(* Logix 5000 Controller export Example_PLC; controller Example_PLC 1769-L32E rev 19.11; software revision 19.01; part 5 of 6 *)
(* tags used below, declared in another part *)
   Incremental : BOOL;   // Position Definition (0=Absolute, 1=Incremental)
   OS_LoadStart : BOOL;
(* AKD_Set_Position, continued *)

ROUTINE Prescan   (* ladder *)
// Prescan
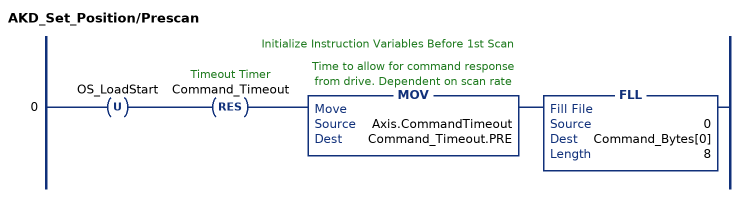
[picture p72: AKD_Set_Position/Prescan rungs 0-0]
   // Initialize Instruction Variables Before 1st Scan
   0: OTU(OS_LoadStart)RES(Command_Timeout)MOV(Axis.CommandTimeout,Command_Timeout.PRE)FLL(0,Command_Bytes[0],8);
END_ROUTINE
END_ADD_ON_INSTRUCTION

ADD_ON_INSTRUCTION AKD_Move_RevB   (* revision 4.1, ExecutePrescan, ExecuteEnableInFalse *)
// Motion Axis Move - Position Move
// Revision note:
// Don't error if Command_Timeout preset is 0
VAR_IN_OUT
   Axis : AKD_Axis; {required}
END_VAR
VAR_INPUT
   Move_Type : SINT; {required}   // Move Type (0=Absolute, 1=Incremental)
   Accel : DINT; {required}   // Acceleration
   Decel : DINT; {required}   // Deceleration
   Speed : DINT; {required}   // Move Speed
   Position : DINT; {required}   // Target Position
END_VAR
VAR_OUTPUT
   DN : BOOL; {access Read Only, visible}   // Command Successfully Initiated
   ER : BOOL; {access Read Only, visible}   // Error
   IP : BOOL; {access Read Only, visible}   // Command in Process
   PC : BOOL; {access Read Only, visible}   // Command Process Complete
END_VAR
VAR
   Step : SINT;   // Sequence Step Number
   Command_Axis_Number : SINT;
   Response_Axis_Number : SINT;
   Set_Accel : AKD_Set_Accel;
   Set_Decel : AKD_Set_Decel;
   Set_Velocity : AKD_Set_Velocity;
   OS_Start_Sequence : BOOL;
   Set_Position : AKD_Set_Position;
   Command_Timeout : TIMER := (PRE := 200);
   Command_Bytes : SINT[64];
   ErrorData : SINT[8];
END_VAR

ROUTINE EnableInFalse   (* ladder *)
// EnableIn_False
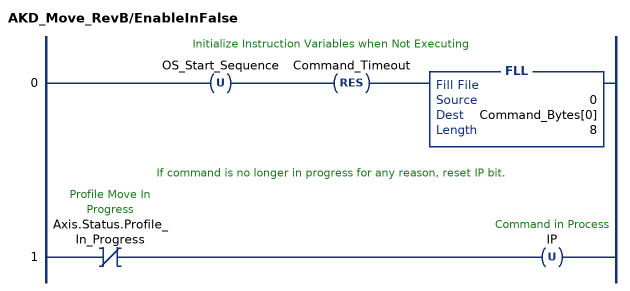
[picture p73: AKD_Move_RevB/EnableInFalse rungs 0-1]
   // Initialize Instruction Variables when Not Executing
   0: OTU(OS_Start_Sequence)RES(Command_Timeout)FLL(0,Command_Bytes[0],8);
   // If command is no longer in progress for any reason, reset IP bit.
   1: XIO(Axis.Status.Profile_In_Progress)OTU(IP);
END_ROUTINE

ROUTINE Logic   (* ladder *)
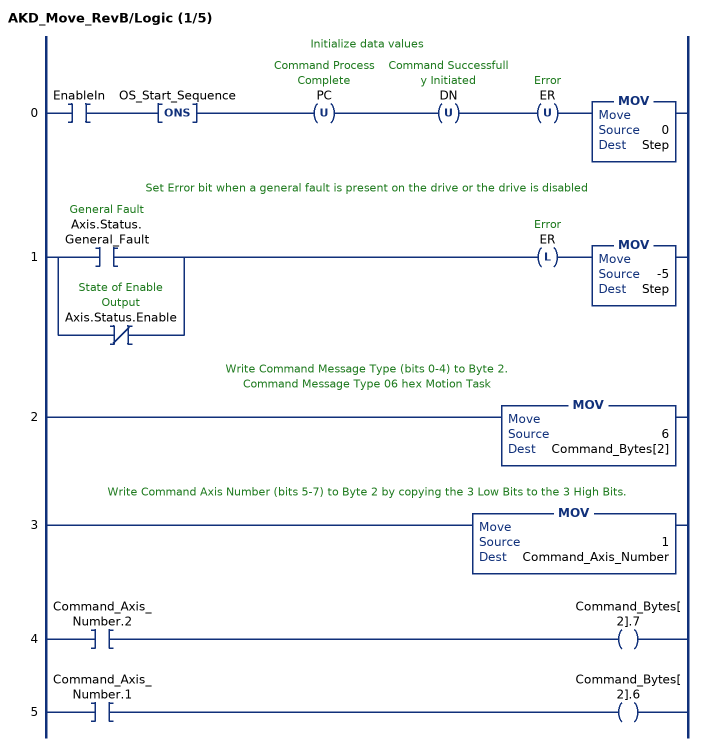
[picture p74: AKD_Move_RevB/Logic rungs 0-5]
   // Initialize data values
   0: XIC(EnableIn)ONS(OS_Start_Sequence)OTU(PC)OTU(DN)OTU(ER)MOV(0,Step);
   // Set Error bit when a general fault is present on the drive or the drive is disabled
   1: [XIC(Axis.Status.General_Fault) ,XIO(Axis.Status.Enable) ]OTL(ER)MOV(-5,Step);
   // Write Command Message Type (bits 0-4) to Byte 2.
   // Command Message Type 06 hex Motion Task
   2: MOV(6,Command_Bytes[2]);
   // Write Command Axis Number (bits 5-7) to Byte 2 by copying the 3 Low Bits to the 3 High Bits.
   3: MOV(1,Command_Axis_Number);
   4: XIC(Command_Axis_Number.2)OTE(Command_Bytes[2].7);
   5: XIC(Command_Axis_Number.1)OTE(Command_Bytes[2].6);
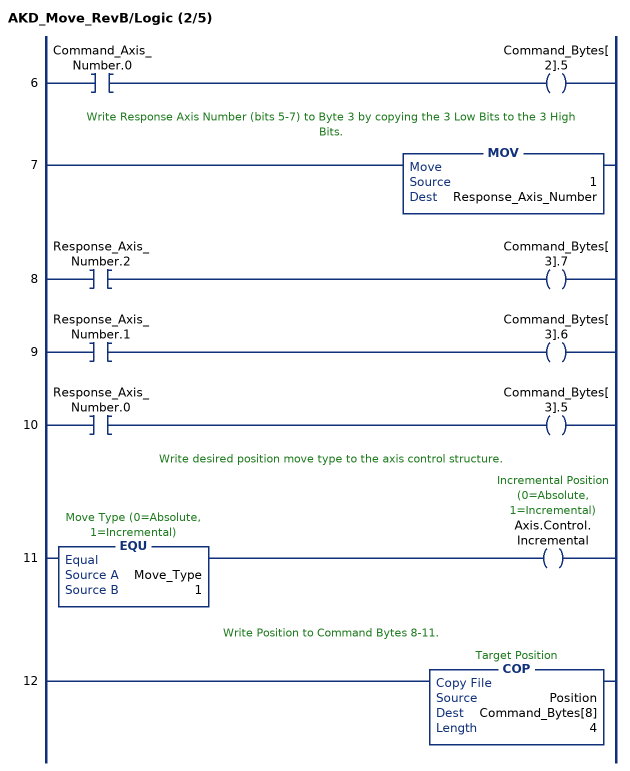
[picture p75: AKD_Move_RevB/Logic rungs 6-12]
   6: XIC(Command_Axis_Number.0)OTE(Command_Bytes[2].5);
   // Write Response Axis Number (bits 5-7) to Byte 3 by copying the 3 Low Bits to the 3 High Bits.
   7: MOV(1,Response_Axis_Number);
   8: XIC(Response_Axis_Number.2)OTE(Command_Bytes[3].7);
   9: XIC(Response_Axis_Number.1)OTE(Command_Bytes[3].6);
   10: XIC(Response_Axis_Number.0)OTE(Command_Bytes[3].5);
   // Write desired position move type to the axis control structure.
   11: EQU(Move_Type,1)OTE(Axis.Control.Incremental);
   // Write Position to Command Bytes 8-11.
   12: COP(Position,Command_Bytes[8],4);
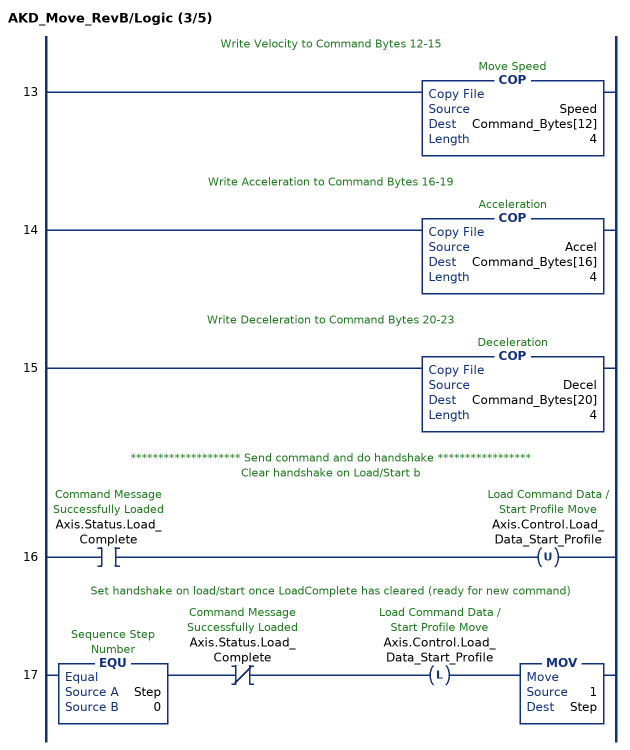
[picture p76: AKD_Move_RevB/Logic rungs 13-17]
   // Write Velocity to Command Bytes 12-15
   13: COP(Speed,Command_Bytes[12],4);
   // Write Acceleration to Command Bytes 16-19
   14: COP(Accel,Command_Bytes[16],4);
   // Write Deceleration to Command Bytes 20-23
   15: COP(Decel,Command_Bytes[20],4);
   // ******************** Send command and do handshake *****************
   // Clear handshake on Load/Start b
   16: XIC(Axis.Status.Load_Complete)OTU(Axis.Control.Load_Data_Start_Profile);
   // Set handshake on load/start once LoadComplete has cleared (ready for new command)
   17: EQU(Step,0)XIO(Axis.Status.Load_Complete)OTL(Axis.Control.Load_Data_Start_Profile)MOV(1,Step);
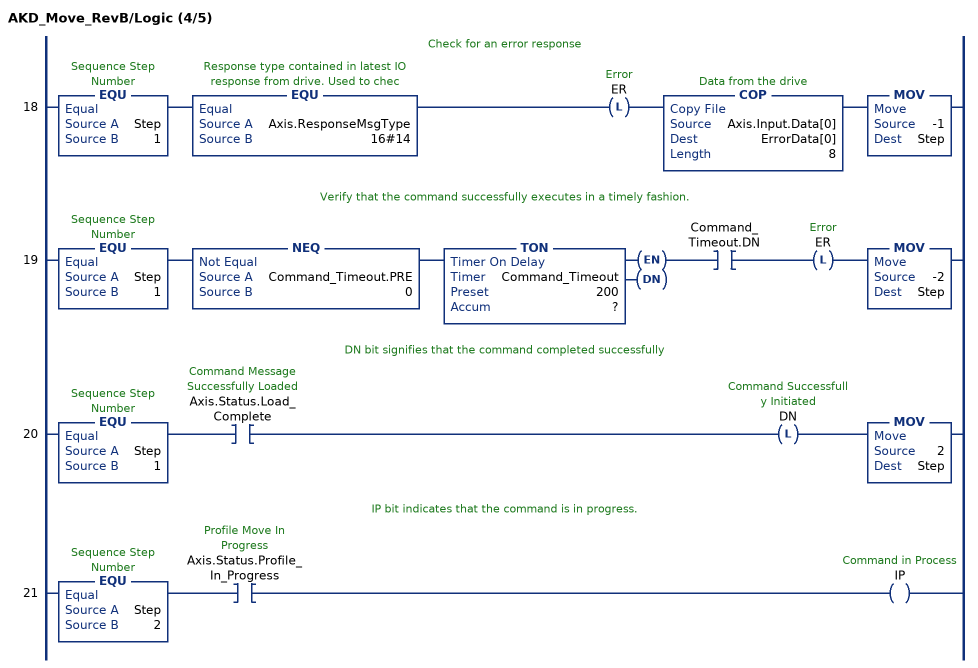
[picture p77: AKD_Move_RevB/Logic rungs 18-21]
   // Check for an error response
   18: EQU(Step,1)EQU(Axis.ResponseMsgType,16#14)OTL(ER)COP(Axis.Input.Data[0],ErrorData[0],8)MOV(-1,Step);
   // Verify that the command successfully executes in a timely fashion.
   19: EQU(Step,1)NEQ(Command_Timeout.PRE,0)TON(Command_Timeout,?,?)XIC(Command_Timeout.DN)OTL(ER)MOV(-2,Step);
   // DN bit signifies that the command completed successfully
   20: EQU(Step,1)XIC(Axis.Status.Load_Complete)OTL(DN)MOV(2,Step);
   // IP bit indicates that the command is in progress.
   21: EQU(Step,2)XIC(Axis.Status.Profile_In_Progress)OTE(IP);
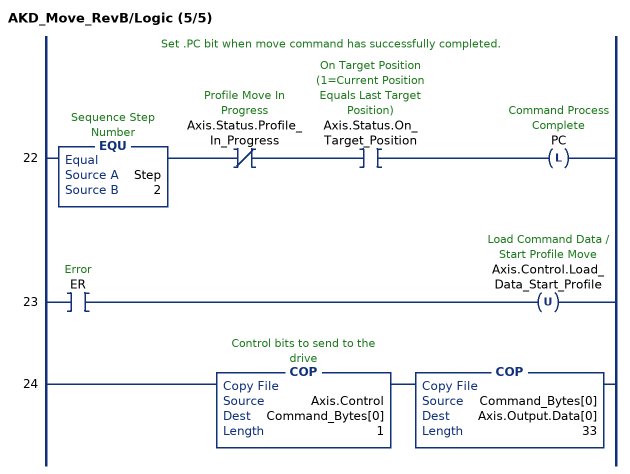
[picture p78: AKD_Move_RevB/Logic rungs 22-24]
   // Set .PC bit when move command has successfully completed.
   22: EQU(Step,2)XIO(Axis.Status.Profile_In_Progress)XIC(Axis.Status.On_Target_Position)OTL(PC);
   23: XIC(ER)OTU(Axis.Control.Load_Data_Start_Profile);
   24: COP(Axis.Control,Command_Bytes[0],1)COP(Command_Bytes[0],Axis.Output.Data[0],33);
END_ROUTINE

ROUTINE Prescan   (* ladder *)
// Prescan
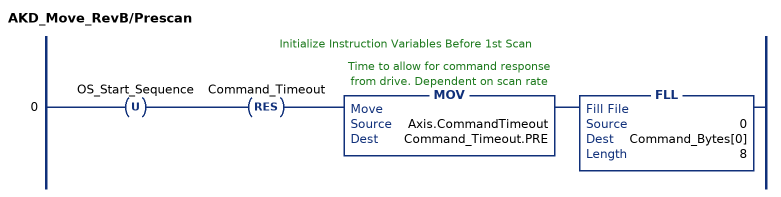
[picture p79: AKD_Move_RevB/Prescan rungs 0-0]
   // Initialize Instruction Variables Before 1st Scan
   0: OTU(OS_Start_Sequence)RES(Command_Timeout)MOV(Axis.CommandTimeout,Command_Timeout.PRE)FLL(0,Command_Bytes[0],8);
END_ROUTINE
END_ADD_ON_INSTRUCTION

ADD_ON_INSTRUCTION AKD_Set_Home_Mode   (* revision 2.0, ExecutePrescan, ExecuteEnableInFalse *)
// Set Homing Mode
VAR_OUTPUT
   DN : BOOL; {access Read Only, visible}   // Command Successful
   ER : BOOL; {access Read Only, visible}   // Error
END_VAR
VAR_IN_OUT
   Axis : AKD_Axis; {required}
END_VAR
VAR_INPUT
   Mode : SINT; {required}   // Home Mode:
END_VAR
VAR
   Command_Bytes : SINT[8];
   Step : DINT;
   Set_Attribute : AKD_Set_Attribute;
END_VAR

ROUTINE EnableInFalse   (* ladder *)
// EnableIn_False
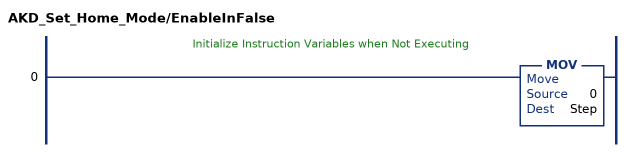
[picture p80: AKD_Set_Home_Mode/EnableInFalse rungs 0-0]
   // Initialize Instruction Variables when Not Executing
   0: MOV(0,Step);
END_ROUTINE

ROUTINE Logic   (* ladder *)
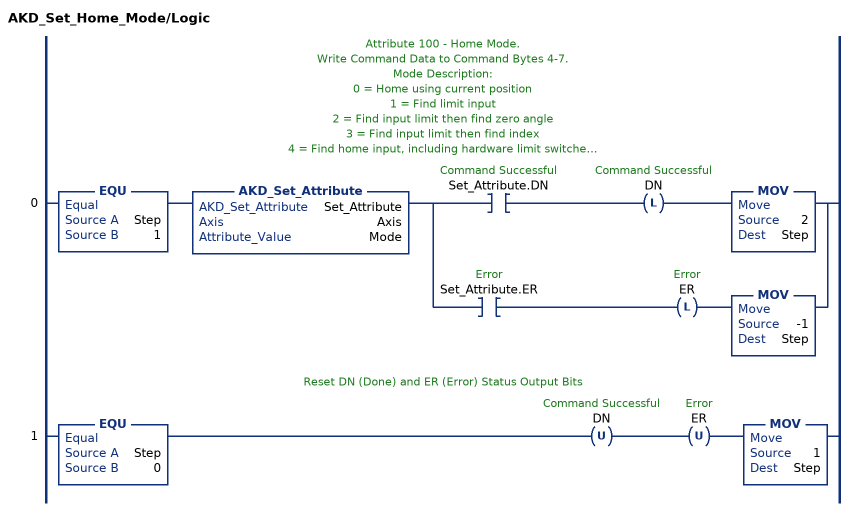
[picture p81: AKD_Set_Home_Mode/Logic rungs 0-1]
   // Attribute 100 - Home Mode.
   // Write Command Data to Command Bytes 4-7.
   // Mode Description:
   // 0 = Home using current position
   // 1 = Find limit input
   // 2 = Find input limit then find zero angle
   // 3 = Find input limit then find index
   // 4 = Find home input, including hardware limit switches
   // 5 = Find home input then find zero angle, including hardware limit switches
   // 6 = Find home input then find index, including hardware limit switches.
   // 7 = Find zero angle
   // 8 = Move until position error exceeded
   // 9 = Move until position error exceeded, then find zero angle
   // 10 = Move until position error exceeded, then find index
   // 11 = Find index signal, without any precondition
   // 12 = Homing to a home-switch, including mechanical stop detection
   0: EQU(Step,1)AKD_Set_Attribute(Set_Attribute,Axis,Mode)[XIC(Set_Attribute.DN) OTL(DN) MOV(2,Step) ,XIC(Set_Attribute.ER) OTL(ER) MOV(-1,Step) ];
   // Reset DN (Done) and ER (Error) Status Output Bits
   1: EQU(Step,0)OTU(DN)OTU(ER)MOV(1,Step);
END_ROUTINE

ROUTINE Prescan   (* ladder *)
// Prescan
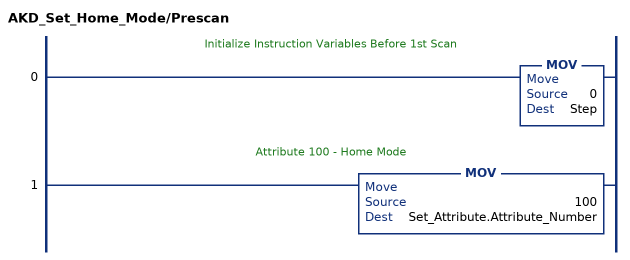
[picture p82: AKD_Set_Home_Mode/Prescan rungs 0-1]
   // Initialize Instruction Variables Before 1st Scan
   0: MOV(0,Step);
   // Attribute 100 - Home Mode
   1: MOV(100,Set_Attribute.Attribute_Number);
END_ROUTINE
END_ADD_ON_INSTRUCTION

ADD_ON_INSTRUCTION AKD_Set_Units   (* revision 2.2, ExecutePrescan, ExecuteEnableInFalse *)
// Set Drive Units for Motion Commands
// Revision note:
// Clean up instruction, especially for error recovery.
VAR_IN_OUT
   Axis : AKD_Axis; {required}
END_VAR
VAR_INPUT
   Units : SINT; {required}   // Drive Units (0=Counts 16 bit)
END_VAR
VAR_OUTPUT
   DN : BOOL; {access Read Only, visible}   // Command Successfully Initiated
   ER : BOOL; {access Read Only, visible}   // Error
END_VAR
VAR
   Set_POSUNIT : AKD_Set_Attribute := (Attribute_Number := 4);
   Set_PROFUNIT : AKD_Set_Attribute := (Attribute_Number := 5);
   Step : SINT;   // Sequence Step Number
   OS_Start_Sequence : BOOL;
   Profile_Ratio : DINT;   // The number of actual feedback counts per second or second2 equal to one velocity or acceleration unit
   Position_Ratio : DINT;   // The number of actual position feedback counts equal to one position unit
   Invalid_Input : BOOL;   // Invalid Units Input
END_VAR

ROUTINE EnableInFalse   (* ladder *)
// EnableIn_False
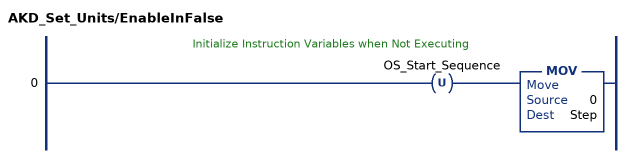
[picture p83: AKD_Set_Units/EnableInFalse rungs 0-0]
   // Initialize Instruction Variables when Not Executing
   0: OTU(OS_Start_Sequence)MOV(0,Step);
END_ROUTINE

ROUTINE Logic   (* ladder *)
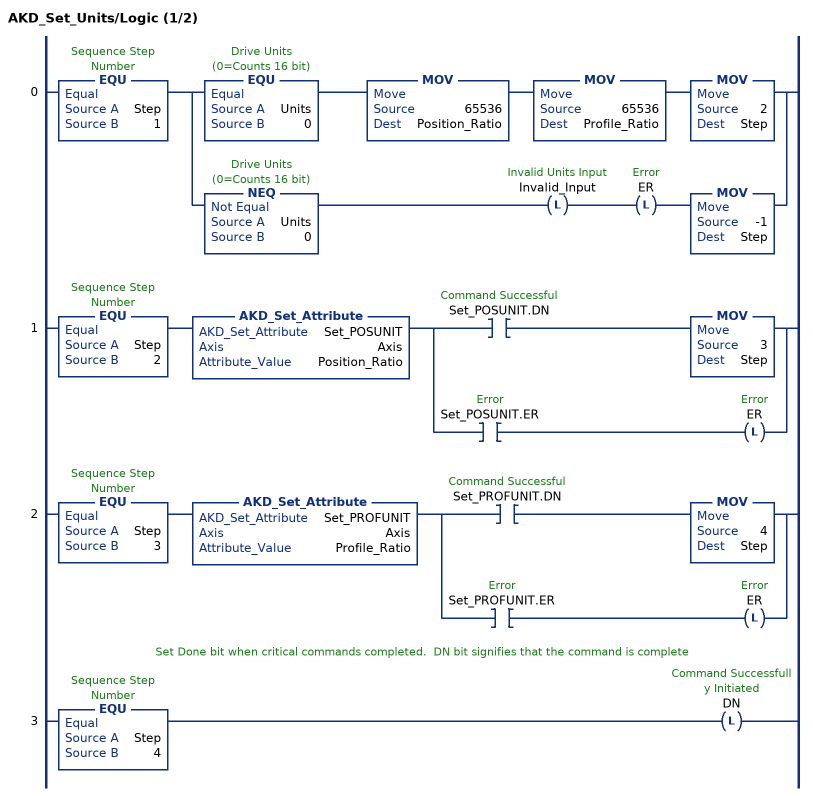
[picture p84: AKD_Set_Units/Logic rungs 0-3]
   0: EQU(Step,1)[EQU(Units,0) MOV(65536,Position_Ratio) MOV(65536,Profile_Ratio) MOV(2,Step) ,NEQ(Units,0) OTL(Invalid_Input) OTL(ER) MOV(-1,Step) ];
   1: EQU(Step,2)AKD_Set_Attribute(Set_POSUNIT,Axis,Position_Ratio)[XIC(Set_POSUNIT.DN) MOV(3,Step) ,XIC(Set_POSUNIT.ER) OTL(ER) ];
   2: EQU(Step,3)AKD_Set_Attribute(Set_PROFUNIT,Axis,Profile_Ratio)[XIC(Set_PROFUNIT.DN) MOV(4,Step) ,XIC(Set_PROFUNIT.ER) OTL(ER) ];
   // Set Done bit when critical commands completed.  DN bit signifies that the command is complete
   3: EQU(Step,4)OTL(DN);
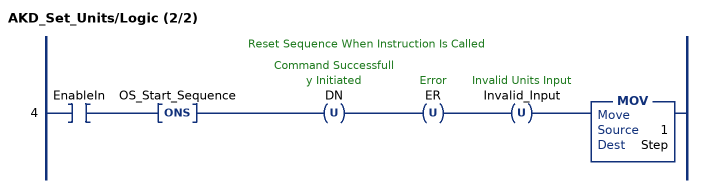
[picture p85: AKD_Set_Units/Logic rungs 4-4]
   // Reset Sequence When Instruction Is Called
   4: XIC(EnableIn)ONS(OS_Start_Sequence)OTU(DN)OTU(ER)OTU(Invalid_Input)MOV(1,Step);
END_ROUTINE

ROUTINE Prescan   (* ladder *)
// Prescan
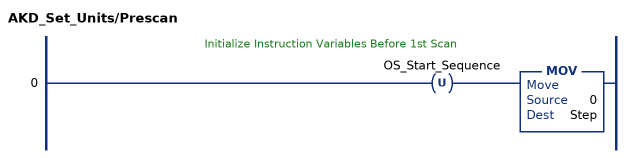
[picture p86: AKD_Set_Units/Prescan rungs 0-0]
   // Initialize Instruction Variables Before 1st Scan
   0: OTU(OS_Start_Sequence)MOV(0,Step);
END_ROUTINE
END_ADD_ON_INSTRUCTION

ADD_ON_INSTRUCTION AKD_Shutdown   (* revision 2.0, ExecutePrescan, ExecuteEnableInFalse *)
// Motion Hard Stop
VAR_OUTPUT
   DN : BOOL; {access Read Only, visible}   // Command Successful
   ER : BOOL; {access Read Only, visible}   // Error
END_VAR
VAR_IN_OUT
   Axis : AKD_Axis; {required}
END_VAR
VAR
   Command_Timeout : TIMER := (PRE := 2000);   // Timeout Timer
END_VAR

ROUTINE EnableInFalse   (* ladder *)
// Enable In False
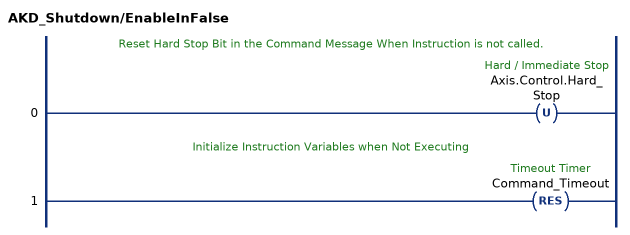
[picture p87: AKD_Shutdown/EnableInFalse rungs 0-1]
   // Reset Hard Stop Bit in the Command Message When Instruction is not called.
   0: OTU(Axis.Control.Hard_Stop);
   // Initialize Instruction Variables when Not Executing
   1: RES(Command_Timeout);
END_ROUTINE

ROUTINE Logic   (* ladder *)
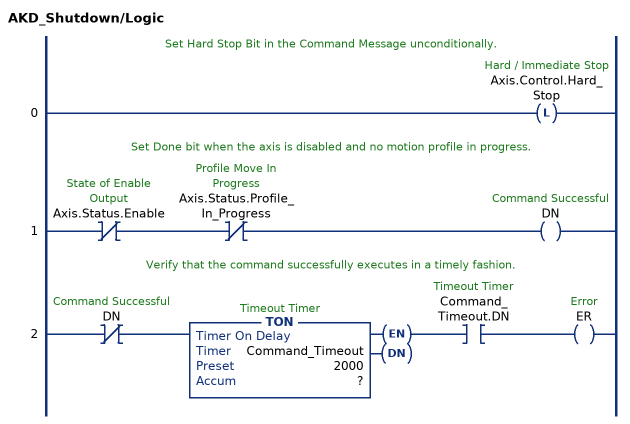
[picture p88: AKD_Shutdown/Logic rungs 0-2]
   // Set Hard Stop Bit in the Command Message unconditionally.
   0: OTL(Axis.Control.Hard_Stop);
   // Set Done bit when the axis is disabled and no motion profile in progress.
   1: XIO(Axis.Status.Enable)XIO(Axis.Status.Profile_In_Progress)OTE(DN);
   // Verify that the command successfully executes in a timely fashion.
   2: XIO(DN)TON(Command_Timeout,?,?)XIC(Command_Timeout.DN)OTE(ER);
END_ROUTINE

ROUTINE Prescan   (* ladder *)
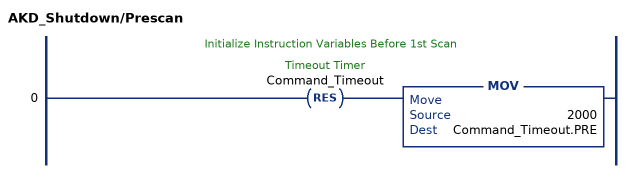
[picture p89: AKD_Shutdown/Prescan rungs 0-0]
   // Initialize Instruction Variables Before 1st Scan
   0: RES(Command_Timeout)MOV(2000,Command_Timeout.PRE);
END_ROUTINE
END_ADD_ON_INSTRUCTION
